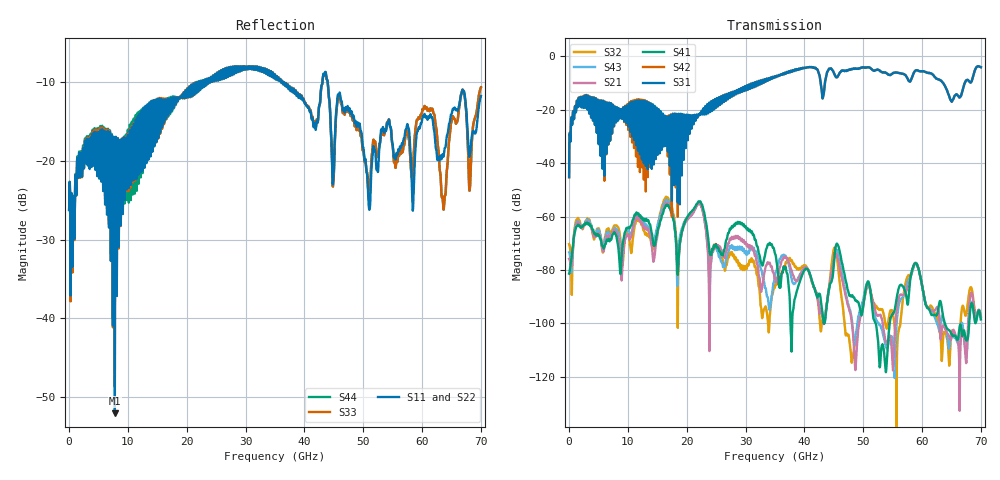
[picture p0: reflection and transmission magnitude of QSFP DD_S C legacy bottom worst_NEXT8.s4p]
! AWR Design Environment (8415) Thu Dec 20 15:51:00 2018
! Document = 'CHANNEL TEST'
! nPorts: 4, nXvals: 7001
# HZ S DB R 50
!Freq DBS11 AngS11 DBS12 AngS12 DBS13 AngS13 DBS14 AngS14
!	DBS21 AngS21 DBS22 AngS22 DBS23 AngS23 DBS24 AngS24
!	DBS31 AngS31 DBS32 AngS32 DBS33 AngS33 DBS34 AngS34
!	DBS41 AngS41 DBS42 AngS42 DBS43 AngS43 DBS44 AngS44
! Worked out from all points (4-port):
!   7000 points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, 10 MHz to 70 GHz, reference 50 ohm
!   strongest paths, dB at 10 MHz, 17.51 GHz, 35.01 GHz, 52.51 GHz, 70 GHz:
!     S31: -45.2, -30.1, -7.6, -5.0, -4.0
!     S42: -45.3, -29.9, -7.6, -5.0, -4.0
!     S41: -81.4, -59.0, -73.9, -106.1, -98.5
!     S21: -75.8, -58.5, -83.4, -96.9, -97.5
!     S43: -73.3, -57.9, -82.2, -99.7, -98.4
!     S32: -70.3, -56.8, -86.3, -94.4, -97.4
!   lowest |S11| = -52.1 dB at 7.78 GHz (marker M1), VSWR 1.00, Z = 49.9 - j0.242 ohm
!   |S11| at or under -10 dB: start of sweep to 21.78 GHz; 36.28 GHz to 43.07 GHz (6.789 GHz wide, 17.1 % of centre); 43.97 GHz to end of sweep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
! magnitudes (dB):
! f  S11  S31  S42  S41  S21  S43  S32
! 10 MHz  -26.3  -45.2  -45.3  -81.4  -75.8  -73.3  -70.3
! 1.65 GHz  -19.9  -15.5  -15.4  -63.5  -62.7  -62.2  -61.2
! 7.78 GHz  -52.1  -18.9  -18.9  -66.0  -65.0  -64.3  -63.3
! 18.58 GHz  -12.0  -23.4  -23.5  -77.4  -78.3  -73.3  -79.5
! 22.14 GHz  -9.9  -21.9  -21.7  -54.4  -55.2  -55.0  -55.0
! 23.95 GHz  -10.0  -20.1  -20.0  -74.1  -83.5  -87.3  -77.0
! 70 GHz  -11.8  -4.0  -4.0  -98.5  -97.5  -98.4  -97.4
